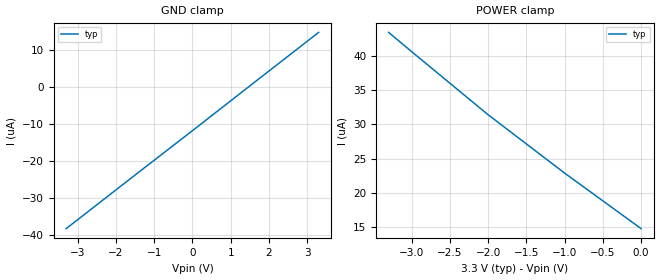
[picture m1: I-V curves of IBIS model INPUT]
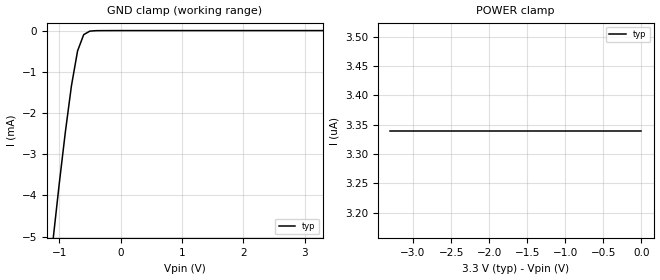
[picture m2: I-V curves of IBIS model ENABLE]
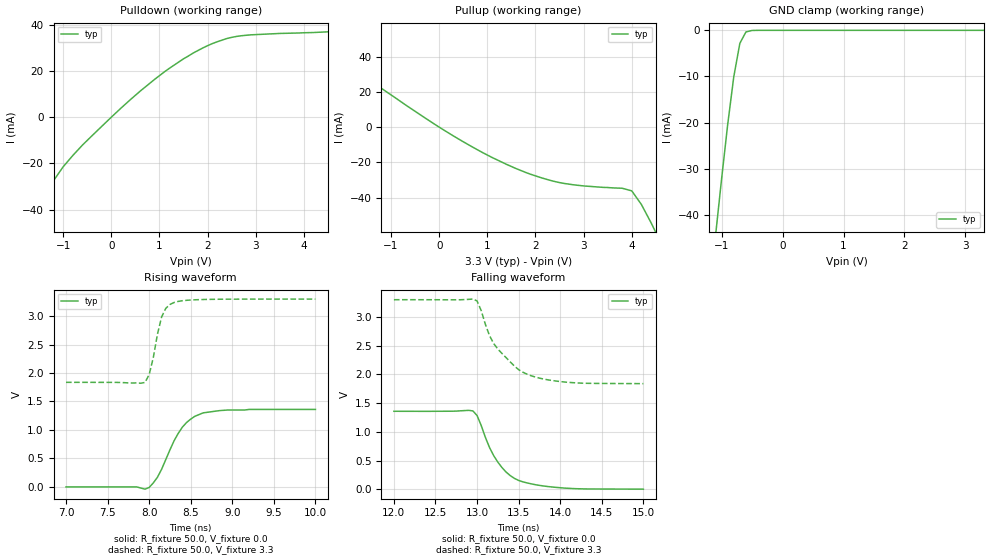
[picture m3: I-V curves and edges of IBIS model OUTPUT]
|   Texas Instruments Incorporated
|   Data Transmissions Products
|   IBIS Model for  SN65LVDT3486B
|   16D SOIC Package
[IBIS Ver]   3.2
[Comment char]   |_char
[File name]   lvt3486b.ibs
[File Rev]   1.0
[Date]   6Nov00
[Source]   File originated at Texas Instruments Incorporated.
   Data Transmission Products Group. All data based on
   Bench Measurements.
[Notes]
[Disclaimer]
(C) Copyright Texas Instruments Incorporated 2000
   All rights reserved
  Texas Instruments Incorporated hereby grants the user of this IBIS
model a non-exclusive, nontransferable license to use this IBIS model
under the following terms.  Before using this IBIS model, the user
should read this license.  If the user does not accept these terms,
the IBIS model should be returned to Texas Instruments within 30 days.
  The user is granted this license only to use the IBIS model and
is not granted rights to sell, load, rent, lease or license the IBIS
model in whole or in part, or in modified form to anyone other than
user.  User may modify the IBIS model to suit its specific applications
but rights to derivative works and such modifications shall belong to
Texas Instruments.
  This IBIS model is provided on an "AS IS" basis and Texas Instruments
makes absolutely no warranty with respect to the information contained
herein.  TEXAS INSTRUMENTS DISCLAIMS AND CUSTOMER WAIVES ALL WARRANTIES,
EXPRESS OR IMPLIED, INCLUDING WARRANTIES OF MERCHANTABILITY OR FITNESS
FOR A PARTICULAR PURPOSE. The entire risk as to quality and performance
is with the Customer. ACCORDINGLY, IN NO EVENT SHALL THE COMPANY BE LIABLE
FOR ANY DAMAGES, WHETHER IN CONTRACT OR TORT,INCLUDING ANY LOST PROFITS
OR OTHER INCIDENTAL, CONSEQUENTIAL, EXEMPLARY, OR PUNITIVE DAMAGES ARISING
OUT OF THE USE OR APPLICATION OF THE IBIS model provided in this package.
Further, Texas Instruments reserves the right to discontinue or make changes
without notice to any product herein to improve reliability, function, or
design. Texas Instruments does not convey any license under patent rights
or any other intellectual property rights, including those of third parties.
Contact Texas Instruments at ATTN:DATA TRANSMISSIONS
[Copyright]   Copyright 2000, Texas Instruments, All Rights Reserved
[Component]   SN65LVDT3486BD
[Manufacturer]  Texas Instruments Incorporated
[Package]
|   typ   min   max
R_pkg   0.035   0.030   0.040
L_pkg   2.181nH   1.231nH   3.257nH
C_pkg   0.322pF   0.163pF   0.546pF
[Pin]   signal_name   model_name   R_pin   L_pin   C_pin
1   1B   INPUT   0.040   3.251n   0.546p
2   1A   INPUT   0.039   2.561n   0.393p
3   1Y   OUTPUT   0.030   1.681n   0.186p
4   1,2EN   ENABLE   0.030   1.231n   0.163p
5   2Y   OUTPUT   0.030   1.231n   0.163p
6   2A   INPUT   0.030   1.681n   0.186p
7   2B   INPUT   0.039   2.564n   0.393p
8   GND   GND   0.040   3.257n   0.545p
9   3B   INPUT   0.040   3.247n   0.546p
10   3A   INPUT   0.039   2.558n   0.394p
11   3Y   OUTPUT   0.030   1.681n   0.187p
12   3,4EN   ENABLE   0.030   1.231n   0.163p
13   4Y   OUTPUT   0.030   1.231n   0.163p
14   4A   INPUT   0.030   1.681n   0.187p
15   4B   INPUT   0.039   2.558n   0.394p
16   VCC   POWER   0.040   3.246n   0.546p
[Diff_pin]   inv_pin   vdiff   tdelay_typ   tdelay_min   tdelay_max
| The 'xA' pin is Diff_pin and the 'xB' pin is the inv_pin
2   1   50mV   0 0 0   | Vth  +/-50mV
6   7   50mV   0 0 0
10   9   50mV   0 0 0
14   15   50mV   0 0 0
| Models and submodels in the file (3): INPUT (Input), ENABLE (Input), OUTPUT (3-state)
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|   Receiver Input  MODEL
[Model]   INPUT
Model_type   Input
|Signals   1A,1B,2A,2B,3A,3B,4A,4B
Vinh = 2.0
Vinl = 0.8
|   typ   min   max
C_comp   1.0pF   NA   NA
|   typ   min   max
[Temperature Range]   25.0   NA   NA
[Voltage range]   3.3V   3.0V   3.6V
[GND_clamp]
|   Voltage   I(typ)   I(min)   I(max)
-3.3V     -38.3uA    NA         NA
-1.3V     -22.2uA    NA         NA
0V        -11.8uA    NA         NA
1.3V      -1.3uA     NA         NA
3.3V      14.8uA     NA         NA
[Power_clamp]
| Note that the[POWER_clamp]voltage table is referenced to Vcc
| and is calculated using Vtable=Vcc - Vmeasured.
|   Voltage   I(typ)   I(min)   I(max)
-3.3V     43.4uA     NA         NA
-3V       40.6uA     NA         NA
-2V       31.4uA     NA         NA
-1V       22.9uA     NA         NA
0V        14.8uA     NA         NA
|   Receiver Enable  MODEL
[Model]   ENABLE
Model_type   Input
|Signals   1,2EN, 3,4EN
Vinh = 2.0
Vinl = 0.8
|   typ   min   max
C_comp   1.0pF   NA   NA
|   typ   min   max
[Temperature Range]   25.0   NA   NA
[Voltage range]   3.3V   3.0V   3.6V
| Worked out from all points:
|   GND clamp passes 1 mA (typ) near -0.76 V on its own axis
[GND_clamp]
|   Voltage   I(typ)   I(min)   I(max)
-3.3V     -43.1mA    NA         NA
-1.1V     -5.08mA    NA         NA
-1V       -3.73mA    NA         NA
-900mV    -2.47mA    NA         NA
-800mV    -1.34mA    NA         NA
-700mV    -493uA     NA         NA
-600mV    -98.5uA    NA         NA
-500mV    -13.3uA    NA         NA
3.3V      3.34pA     NA         NA
[Power_clamp]
| Note that the[POWER_clamp]voltage table is referenced to Vcc
| and is calculated using Vtable=Vcc - Vmeasured.
|   Voltage   I(typ)   I(min)   I(max)
-3.3V     3.34uA     NA         NA
-2.7V     3.34uA     NA         NA
-2V       3.34uA     NA         NA
-800mV    3.34uA     NA         NA
0V        3.34uA     NA         NA
|   Receiver Output  MODEL
[Model]   OUTPUT
Model_type   3-state
| Signals   1Y,2Y,3Y,4Y
Vmeas = 1.5V   |Reference voltage for timing measurements
Cref = 8pF   |Timing specification test load capacitance value
Vref = 0   |Timing specification test load voltage; GND
| variable   typ   min   max
C_comp   1.0pF   NA   NA
|   typ   min   max
[Temperature Range]   25.0   NA   NA
[Voltage range]   3.3V   3.0V   3.6V
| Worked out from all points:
|   slope of the pulldown table from 0 to 0.495 V, typ, clamps not added: 52.7 ohm
|   slope of the pullup table from 0 to 0.495 V, typ, clamps not added: 60.3 ohm
|   GND clamp passes 1 mA (typ) near -0.63 V on its own axis
|   rising waveform, R_fixture 50.0, V_fixture 0.0: 20-80 % time 287ps typ, NA min, NA max; typ from 0 V to 1.36 V
|   falling waveform, R_fixture 50.0, V_fixture 0.0: 20-80 % time 315ps typ, NA min, NA max; typ from 1.36 V to 0.004 V
|   rising waveform, R_fixture 50.0, V_fixture 3.3: 20-80 % time 131ps typ, NA min, NA max; typ from 1.84 V to 3.3 V
|   falling waveform, R_fixture 50.0, V_fixture 3.3: 20-80 % time 389ps typ, NA min, NA max; typ from 3.3 V to 1.84 V
[Pulldown]
|   Voltage   I(typ)   I(min)   I(max)
-3.3V     -150mA     NA         NA
-1.6V     -47.9mA    NA         NA
-1.2V     -27.5mA    NA         NA
-1V       -21.5mA    NA         NA
-600mV    -12.1mA    NA         NA
200mV     3.91mA     NA         NA
900mV     16.4mA     NA         NA
1.5V      25.3mA     NA         NA
2.1V      31.9mA     NA         NA
2.5V      34.6mA     NA         NA
2.9V      35.7mA     NA         NA
6.6V      39.1mA     NA         NA
[Pullup]
|   Voltage   I(typ)   I(min)   I(max)
| Note that the[Pullup]voltage table is referenced to Vcc
| and is calculated using Vtable=Vcc - Vmeasured.
-3.3V     61mA       NA         NA
-3.1V     57.2mA     NA         NA
-3V       55.4mA     NA         NA
100mV     -1.72mA    NA         NA
900mV     -14.4mA    NA         NA
1.6V      -23.5mA    NA         NA
2.5V      -31.4mA    NA         NA
4V        -36.1mA    NA         NA
4.2V      -43.8mA    NA         NA
4.4V      -54.1mA    NA         NA
4.6V      -65.3mA    NA         NA
6.6V      -187mA     NA         NA
| Output in High Impedance (off)
[GND_clamp]
|   Voltage   I(typ)   I(min)   I(max)
-3.3V     -347mA     NA         NA
-1.1V     -44.7mA    NA         NA
-1V       -32.3mA    NA         NA
-900mV    -20.5mA    NA         NA
-800mV    -10.1mA    NA         NA
-700mV    -2.82mA    NA         NA
-600mV    -350uA     NA         NA
-500mV    -29.4uA    NA         NA
-400mV    -1.91uA    NA         NA
3.3V      426pA      NA         NA
[POWER_clamp]
|   Voltage   I(typ)   I(min)   I(max)
| Note that the [POWER_clamp] voltage table is referenced to Vcc
| and is calculated using Vtable = Vcc - Vmeasured.
| Outputs in Tri-state.
-3.3V     0A         NA         NA
0V        0A         NA         NA
[Ramp]
|   typ   min   max
dV/dt_r   0.815V/389ps   NA   NA
dV/dt_f   0.880V/285ps   NA   NA
R_load = 50
[Rising Waveform]
R_fixture = 50.0
V_fixture = 0.0
C_fixture = 0p
L_fixture = 0n
|   V(typ)   V(min)   V(max)
7ns       0V         NA         NA
7.95ns    -40mV      NA         NA
8ns       -10mV      NA         NA
8.1ns     170mV      NA         NA
8.3ns     810mV      NA         NA
8.4ns     1.05V      NA         NA
8.5ns     1.19V      NA         NA
8.65ns    1.3V       NA         NA
8.95ns    1.35V      NA         NA
10ns      1.36V      NA         NA
[Falling Waveform]
R_fixture = 50.0
V_fixture = 0.0
C_fixture = 0p
L_fixture = 0n
|   V(typ)   V(min)   V(max)
12ns      1.359V     NA         NA
12.95ns   1.365V     NA         NA
13ns      1.285V     NA         NA
13.15ns   728mV      NA         NA
13.25ns   474mV      NA         NA
13.4ns    239mV      NA         NA
13.55ns   132mV      NA         NA
13.8ns    59mV       NA         NA
14.05ns   23mV       NA         NA
15ns      4mV        NA         NA
[Rising Waveform]
R_fixture = 50.0
V_fixture = 3.3
C_fixture = 0p
L_fixture = 0n
|   V(typ)   V(min)   V(max)
7ns       1.836V     NA         NA
7.95ns    1.834V     NA         NA
8ns       1.971V     NA         NA
8.05ns    2.27V      NA         NA
8.1ns     2.682V     NA         NA
8.15ns    2.984V     NA         NA
8.2ns     3.135V     NA         NA
8.3ns     3.238V     NA         NA
8.7ns     3.292V     NA         NA
10ns      3.298V     NA         NA
[Falling Waveform]
R_fixture = 50.0
V_fixture = 3.3
C_fixture = 0p
L_fixture = 0n
|   V(typ)   V(min)   V(max)
12ns      3.299V     NA         NA
12.95ns   3.311V     NA         NA
13ns      3.279V     NA         NA
13.05ns   3.109V     NA         NA
13.15ns   2.674V     NA         NA
13.2ns    2.537V     NA         NA
13.45ns   2.144V     NA         NA
13.65ns   1.977V     NA         NA
14.1ns    1.862V     NA         NA
15ns      1.84V      NA         NA
